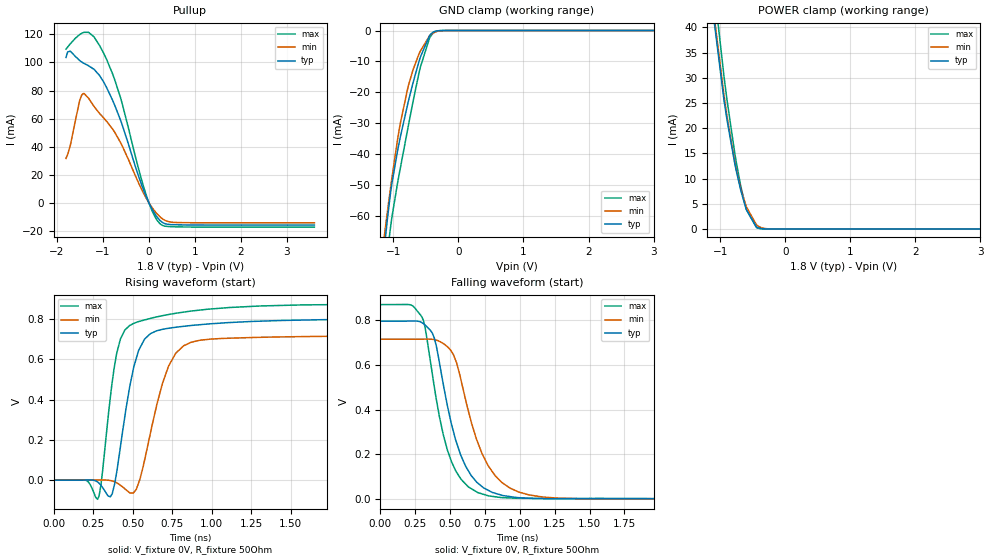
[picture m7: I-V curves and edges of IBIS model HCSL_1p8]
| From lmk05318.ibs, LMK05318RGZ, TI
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|   HCSL_1p8 Model
[Model]   HCSL_1p8
Model_type   Open_source
Polarity   Non-Inverting
Vmeas = 0.405
Vref = 0
Cref = 2pF
Rref = 50
|   typ   min   max
C_comp   1.5263E-12   1.43105E-12   1.63546E-12
| Where nom  PVT is Nominal Process, 1.8V, 27C
|   Fast PVT is Strong Process,  1.9V, -40C
|   Slow PVT is Weak Process,   1.7V, 125C
[Voltage Range]   1.8   1.7   1.9
|Junction Temperature
[Temperature Range]   27   125   -40
[Pullup Reference]   1.8   1.7   1.9
[Pulldown Reference]   0   0   0
[Power Clamp Reference]   1.8   1.7   1.9
[GND Clamp Reference]   0   0   0
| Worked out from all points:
|   slope of the pullup table from 0 to 0.27 V, typ, clamps not added: 20 ohm
|   GND clamp passes 1 mA (typ) near -0.42 V on its own axis
|   POWER clamp passes 1 mA (typ) near -0.47 V on its own axis
|   falling waveform, V_fixture 0V, R_fixture 50Ohm: 20-80 % time 187ps typ, 218ps min, 167ps max; typ from 0.794 V to 0 V
|   rising waveform, V_fixture 0V, R_fixture 50Ohm: 20-80 % time 113ps typ, 143ps min, 93.7ps max; typ from -0.001 V to 0.794 V
[GND Clamp]
|   Voltage   I(typ)   I(min)   I(max)
-1.8V     -227.5mA   -244.3mA   -293.8mA
-1.125V   -67.81mA   -64.27mA   -79.09mA
-1.114V   -65.59mA   -62.48mA   -76.82mA
-1.093V   -61.33mA   -58.94mA   -72.53mA
-1.049V   -53.68mA   -52.02mA   -64.8mA
-909mV    -36.18mA   -32mA      -46.42mA
-768.6mV  -22.88mA   -17.82mA   -30.77mA
-585mV    -8.613mA   -6.634mA   -11.87mA
-444.6mV  -1.694mA   -1.777mA   -2.489mA
-385.2mV  -510.7uA   -772.5uA   -830.7uA
-217.8mV  -3.668uA   -26.55uA   -3.583uA
3.6V      0A         0A         0A
[Pullup]
|   Voltage   I(typ)   I(min)   I(max)
-1.8V     103.6mA    31.57mA    109.5mA
-1.708V   108.1mA    40.47mA    113.2mA
-1.503V   101.4mA    72.74mA    119.9mA
-1.406V   99.32mA    77.86mA    121.5mA
-1.184V   94.93mA    68.45mA    118mA
-790.2mV  73.34mA    52.7mA     92.19mA
-590.4mV  56.79mA    41.42mA    72.27mA
-61.2mV   4.727mA    3.551mA    6.017mA
111.6mV   -6.869mA   -5.232mA   -8.554mA
268.2mV   -13.35mA   -10.74mA   -15.61mA
613.8mV   -15.77mA   -14.14mA   -17.24mA
3.6V      -15.97mA   -14.34mA   -17.45mA
[POWER Clamp]
|   Voltage   I(typ)   I(min)   I(max)
-1.8V     167.1mA    290.8mA    175.6mA
-1.103V   42.32mA    43.41mA    48.96mA
-941.4mV  25.56mA    26.6mA     30.29mA
-892.8mV  21.47mA    22.2mA     25.41mA
-774mV    12.9mA     13.11mA    14.91mA
-752.4mV  11.54mA    11.74mA    13.24mA
-682.2mV  7.588mA    7.904mA    8.398mA
-595.8mV  3.783mA    4.344mA    3.83mA
-444.6mV  459.2uA    875.5uA    303.4uA
-352.8mV  57.32uA    198.5uA    23.38uA
-217.8mV  991nA      11.87uA    112.9nA
3.6V      0A         0A         0A
[Ramp]
R_load = 50
|   typ   min   max
dV/dt_r   0.476754/1.12889e-10   0.42843/1.42833e-10   0.520992/9.36747e-11
dV/dt_f   0.476755/1.8726e-10   0.428416/2.18155e-10   0.521011/1.67144e-10
[Falling Waveform]
V_fixture = 0V
V_fixture_min = 0V
V_fixture_max = 0V
R_fixture = 50Ohm
C_fixture = 0F
|   Time   V(typ)   V(min)   V(max)
0s        794.2mV    713.8mV    867.9mV
221.1ps   794.5mV    713.7mV    866.1mV
299.6ps   787mV      713.8mV    811.3mV
386.9ps   719.1mV    711.8mV    500.8mV
503.9ps   350.7mV    665mV      178mV
611.9ps   146.4mV    441.5mV    67.38mV
773.7ps   39.79mV    148.9mV    15.26mV
928.2ps   12mV       50.03mV    5.698mV
1.277ns   2.076mV    4.691mV    3.694mV
5ns       -417.2uV   -195.3uV   -407.7uV
[Rising Waveform]
V_fixture = 0V
V_fixture_min = 0V
V_fixture_max = 0V
R_fixture = 50Ohm
C_fixture = 0F
|   Time   V(typ)   V(min)   V(max)
0s        -567.8uV   -320.7uV   -592.1uV
203.3ps   -63.4uV    131.1uV    -823.4uV
278.5ps   -9.616mV   298.4uV    -95.87mV
359ps     -83.78mV   -2.374mV   408.2mV
422.9ps   163.8mV    -25.76mV   700.6mV
523.6ps   605.1mV    -45.94mV   783.4mV
631.5ps   734.2mV    299.4mV    807.1mV
773ps     759.2mV    630.1mV    828.9mV
928.2ps   772.1mV    695mV      844.8mV
5ns       794mV      713.7mV    867.7mV
